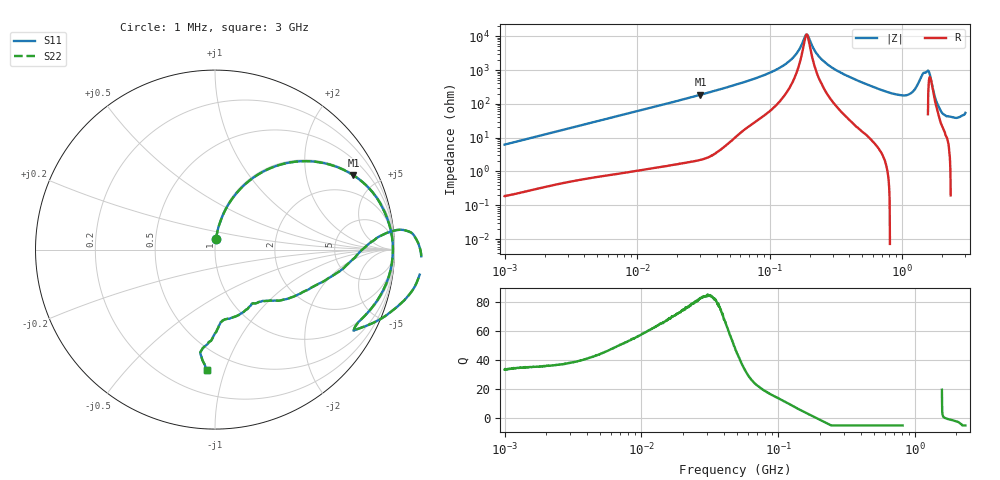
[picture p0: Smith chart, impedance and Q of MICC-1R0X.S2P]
!s-Parameter Generated by FASTRON Sdn. Bhd.
!FASTRON P/N : MICC-1R0X
!Keysight Technologies,E4991B,MY54100416,A.01.15
!Date: Fri Aug 28 09:14:49 2026
!Version  : Rev00 Fri Aug 28 09:14:49 2026
!Data & Calibration Information:
!PortZ  Port1:50+j0  Port2:50+j0
!When reading, reference impedance value at option line is always used.
!Remarks : This data is being provided solely for informational purposes.
!Freq	S11	S21	S12	S22
# Hz S dB R 50
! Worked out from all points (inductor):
!   1601 points, 1 MHz to 3 GHz, reference 50 ohm
!   read as one part in series: L = 988 nH near 1.041 MHz
!   highest Q = 83.7 at 30.05 MHz (marker M1), where L = 980 nH
!   self-resonance near 189.5 MHz
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1000000  -24.14 84.7  -0.03 -3.6  -0.03 -3.6  -24.14 84.7
3804036  -12.97 75.6  -0.28 -13.0  -0.28 -13.0  -12.97 75.6
7588332  -7.66 64.4  -0.89 -24.5  -0.89 -24.5  -7.66 64.4
1.447069e7  -3.70 48.3  -2.53 -40.8  -2.53 -40.8  -3.70 48.3
3.00453e7  -1.16 28.2  -6.50 -61.1  -6.50 -61.1  -1.16 28.2
5.477226e7  -0.38 15.3  -11.56 -73.1  -11.56 -73.1  -0.38 15.3
1.295243e8  -0.10 3.9  -23.19 -78.9  -23.19 -78.9  -0.10 3.9
1.590202e8  -0.08 1.8  -29.64 -72.8  -29.64 -72.8  -0.08 1.8
1.88513e8  -0.08 0.1  -40.92 -11.1  -40.92 -11.1  -0.08 0.1
2.083556e8  -0.08 -0.9  -34.70 60.3  -34.70 60.3  -0.08 -0.9
2.421036e8  -0.09 -2.5  -26.98 75.9  -26.98 75.9  -0.09 -2.5
3.093771e8  -0.11 -5.4  -20.55 79.3  -20.55 79.3  -0.11 -5.4
7.925923e8  -0.85 -24.8  -7.56 65.1  -7.56 65.1  -0.85 -24.8
1.165162e9  -0.52 -26.9  -6.84 69.4  -6.84 69.4  -0.52 -26.9
1.395152e9  1.24 -5.3  -14.76 144.0  -14.76 144.0  1.24 -5.3
1.565327e9  -0.09 5.9  -19.72 -81.1  -19.72 -81.1  -0.09 5.9
1.629261e9  -1.18 2.8  -17.38 -18.7  -17.38 -18.7  -1.18 2.8
1.791767e9  -4.29 -18.0  -6.73 24.2  -6.73 24.2  -4.29 -18.0
1.931433e9  -6.66 -37.4  -3.21 24.1  -3.21 24.1  -6.66 -37.4
2.134733e9  -8.64 -54.1  -1.53 20.9  -1.53 20.9  -8.64 -54.1
2.543347e9  -8.08 -82.6  0.23 22.4  0.23 22.4  -8.08 -82.6
3e9  -3.44 -94.0  1.90 32.7  1.90 32.7  -3.44 -94.0
